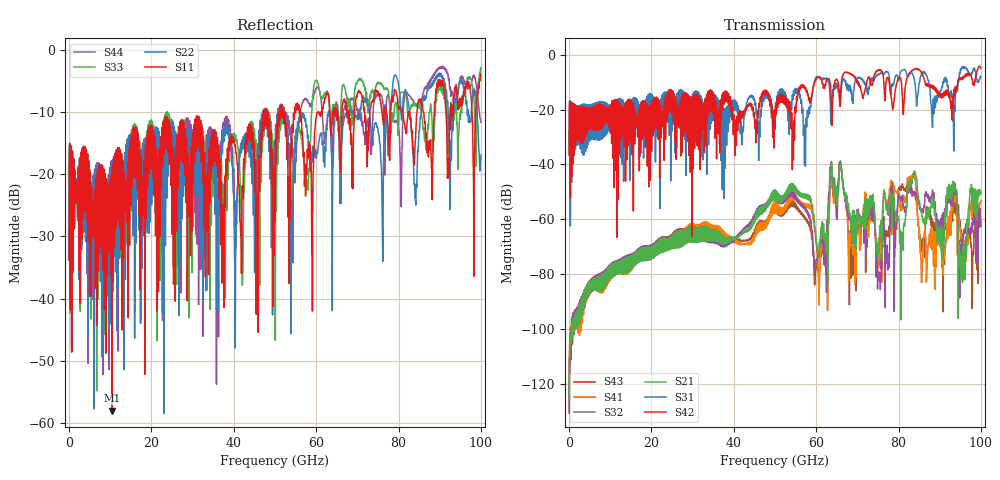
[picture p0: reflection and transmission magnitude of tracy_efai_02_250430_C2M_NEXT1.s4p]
!! PART DESCRIPTION: TE 224G+ VSR Channel- Chip to module, IO connector to CPC(Co-packaged connector) through over the board cable
!! CHANNEL DESCRIPTION: Module trace -> Mated IO 224G+ Connector -> Internal Cable Termination -> 30AWG 300mm Cable -> Cable
!!  termination + CPC connector(No footprint or package included)
!! MODEL REVISION:  Rev 3, Created on April 25, 2025
!! MODEL STATUS: Development
!! MODEL GEOMETRY: 8 Pair Channel
!! MODEL FREQUENCY RANGE: 0 GHz to 100 GHz in 10.00 MHz frequency steps
!! MODEL EDGE RATE LIMITATION: 5ps (Using conservative 0.5/Fmax rule of thumb)
!! PORT DEFINITIONS:
!! Port  1  ----->  Module Side  -->  Host Side, A Row  <-----  Port  2
!! Port  3  ----->  Module Side  -->  Host Side, A Row  <-----  Port  4
# GHz S MA R 45
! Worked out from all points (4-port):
!   10000 points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, 10 MHz to 100 GHz, reference 45 ohm
!   strongest paths, dB at 10 MHz, 25.01 GHz, 50.01 GHz, 75.01 GHz, 100 GHz:
!     S42: -36.5, -18.7, -26.9, -5.6, -4.8
!     S31: -36.5, -27.8, -27.1, -7.4, -8.0
!     S21: -125.2, -70.6, -49.8, -73.2, -50.0
!     S32: -126.0, -70.1, -50.3, -79.5, -61.0
!     S41: -123.9, -70.0, -54.3, -73.5, -53.2
!     S43: -130.8, -69.5, -54.9, -75.5, -62.5
!   lowest |S11| = -58.0 dB at 10.38 GHz (marker M1), VSWR 1.00, Z = 45 + j0.107 ohm
!   |S11| at or under -10 dB: start of sweep to 47.36 GHz; 48.09 GHz to 51.06 GHz (2.963 GHz wide, 5.98 % of centre); 56.14 GHz to 60.39 GHz (4.253 GHz wide, 7.3 % of centre)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
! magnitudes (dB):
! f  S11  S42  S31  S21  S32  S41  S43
! 10 MHz  -33.8  -36.5  -36.5  -125.2  -126.0  -123.9  -130.8
! 10.38 GHz  -58.0  -22.5  -23.2  -76.3  -75.9  -76.6  -76.3
! 60.44 GHz  -10.0  -8.2  -8.0  -72.3  -73.6  -76.3  -78.8
! 65.88 GHz  -19.2  -14.8  -18.1  -39.6  -38.9  -39.3  -38.8
! 75.36 GHz  -7.4  -5.5  -7.1  -66.6  -81.4  -74.1  -75.2
! 82.36 GHz  -10.2  -7.5  -7.9  -48.6  -49.6  -46.2  -46.4
! 100 GHz  -4.0  -4.8  -8.0  -50.0  -61.0  -53.2  -62.5
